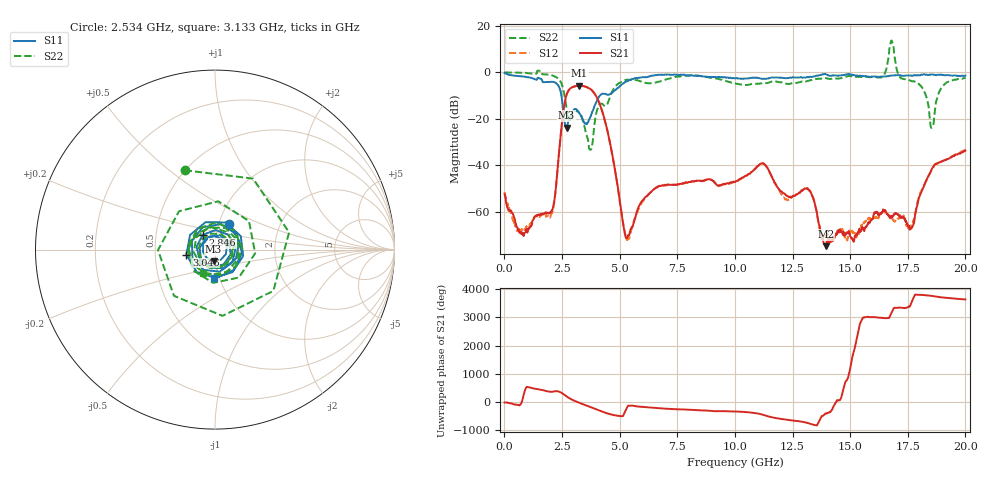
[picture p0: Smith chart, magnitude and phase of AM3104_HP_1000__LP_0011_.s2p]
!Created with skrf (http://scikit-rf.org).
# Hz S RI R 50.0
!freq ReS11 ImS11 ReS21 ImS21 ReS12 ImS12 ReS22 ImS22
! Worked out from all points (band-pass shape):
!   1601 points, 10 MHz to 20 GHz, reference 50 ohm
!   highest |S21| = -5.79 dB at 3.246 GHz (marker M1); lowest = -74.8 dB at 13.95 GHz (marker M2)
!   |S21| within 3 dB of the highest: 2.733 GHz to 3.886 GHz (1.153 GHz wide, 34.9 % of centre)
!   lowest |S11| = -23.8 dB at 2.696 GHz (marker M3), VSWR 1.14, Z = 48.8 - j6.3 ohm
!   |S11| at or under -10 dB: 2.474 GHz to 4.15 GHz (1.676 GHz wide, 50.6 % of centre)
!   |S22| runs from -33.3 to 13.7 dB; largest |S21 - S12| = 0.027
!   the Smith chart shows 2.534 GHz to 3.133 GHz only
!   S11 on the Smith chart (normalised r, x): 2.534 GHz: 1.12, +0.33; 2.846 GHz: 0.86, +0.14; 3.046 GHz: 0.72, -0.04; 3.133 GHz: 0.94, -0.31
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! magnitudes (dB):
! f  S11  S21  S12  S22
! 10 MHz  -0.4  -52.5  -51.6  0.0
! 747.1 MHz  -1.7  -69.0  -67.9  -0.3
! 1.997 GHz  -4.1  -60.4  -62.4  -1.2
! 2.534 GHz  -15.7  -18.7  -18.8  -6.5
! 2.696 GHz  -23.8  -9.8  -9.7  -15.5
! 2.846 GHz  -19.4  -7.1  -7.1  -20.6
! 3.046 GHz  -15.8  -6.1  -6.1  -16.4
! 3.133 GHz  -16.0  -5.9  -5.9  -16.8
! 3.246 GHz  -17.5  -5.8  -5.9  -17.5
! 3.346 GHz  -19.3  -5.9  -5.9  -18.7
! 3.746 GHz  -19.0  -7.3  -7.4  -33.3
! 4.27 GHz  -9.2  -17.6  -17.6  -13.8
! 5.32 GHz  -3.9  -71.4  -71.7  -3.2
! 6.682 GHz  -1.1  -49.1  -49.0  -4.1
! 10.01 GHz  -2.6  -47.2  -47.2  -4.8
! 13.34 GHz  -2.0  -52.9  -52.8  -3.4
! 13.95 GHz  -0.9  -74.8  -70.3  -2.6
! 16.68 GHz  -1.6  -62.1  -61.5  7.2
! 17.68 GHz  -1.5  -66.8  -66.2  -3.8
! 18.54 GHz  -0.9  -41.7  -41.9  -23.9
! 19 GHz  -1.2  -38.3  -38.2  -6.2
! 20 GHz  -1.5  -33.7  -33.5  -2.5
